| Teraspeed (R) Labs.
| http://www.teraspeed.com
[IBIS Ver]   3.2
[Comment Char] |_char
[File Name]   lm98620.ibs
[File Rev]   3.0
[Source]  Teraspeed (R) Labs.
[Date]   02-17-2009
[Notes]   Quality Check of this IBIS model: Model Passes IBIS Check
   Model parses into ICX IS. Simulation done with Hyperlynx.
   1. MIN TYP MAX information is based on Temprature and Voltage
   characteristics only.
   2. Package data measured using Tektronix IConnect Software.
[Disclaimer]
|(C) Copyright National Semiconductor Corporation 2009
|   All rights reserved
|   National Semiconductor Corporation hereby grants
|the user of this IBIS model a non-exclusive, nontransferable
|license to use this IBIS model under the following terms.
|Before using this IBIS model, the user should read this
|license.  If the user does not accept these terms,  the
|IBIS model should be returned to National within 30 days.
|   The user is granted this license only to use the
|IBIS model and is not granted rights to sell, load, rent,
|lease or license the IBIS model in whole or in part, or in
|modified form to anyone other than user. User may modify
|the IBIS model to suit its specific applications but rights
|to derivative works and such modifications shall belong to
|National.
|   This IBIS model is provided on an "AS IS" basis and
|National makes absolutely no warranty with respect to the
|information contained herein.NATIONAL DISCLAIMS AND CUSTOMER
|WAIVES ALL WARRANTIES, EXPRESS OR IMPLIED, INCLUDING
|WARRANTIES OF MERCHANTABILITY OR FITNESS FOR A PARTICULAR
|PURPOSE. The entire risk as to quality and performance is
|with the Customer. ACCORDINGLY, IN NO EVENT SHALL THE
|COMPANY BE LIABLE FOR ANY DAMAGES, WHETHER IN CONTRACT OR
|TORT,INCLUDING ANY LOST PROFITS OR OTHER INCIDENTAL,
|CONSEQUENTIAL, EXEMPLARY, OR PUNITIVE DAMAGES ARISING OUT
|OF THE USE OR APPLICATION OF THE IBIS model provided in
|this package.Further, National reserves the right to make
|changes without notice to any product herein to improve
|reliability, function, or design. National does not convey
|any license under patent rights or any other intellectual
|property rights, including those of third parties.
|   National is not obligated to provide maintenance or support
|for the licensed IBIS model.
| Use: Teraspeed (R) Labs has licensed Teraspeed (R) AccuModel (tm)
| IBIS models to specific integrated circuit suppliers ("IC Vendors")
| for use and distribution as  follows: Each IC Vendor may use IBIS
| Models, and distribute them to IC Vendor's customers to use solely
| for developing printed circuit board designs. Users of this model may
| modify the IBIS model to suit its specific applications but
| rights to derivative works and such modifications shall belong
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[Copyright]
| This file is the legal property of National Semiconductor and
| Teraspeed Copyright(c) 2009.
| All other rights are reserved.
[Component]   LM98620
[Manufacturer] National Semiconductor
[Package]
| variable   typ   min   max
R_pkg  1.848E-02   1.490E-02   2.216E-02
L_pkg  1.664E-09   1.340E-09   1.990E-09
C_pkg  4.630E-13   3.720E-13   5.590E-13
[Pin] signal_name  model_name  R_pin  L_pin C_pin
1   SHD/HOLD   in_gen   2.216E-02  1.990E-09  5.590E-13
2   VDDD   POWER   2.134E-02  1.920E-09  5.370E-13
3   VSSD   GND   2.060E-02  1.850E-09  5.150E-13
4   CLPIN   in_gen   1.970E-02  1.780E-09  4.930E-13
5   BLKCLP   in_pd   1.890E-02  1.700E-09  4.720E-13
6   AGC_ONB   in_pu   1.800E-02  1.620E-09  4.510E-13
7   OVPB   in_gen   1.720E-02  1.550E-09  4.300E-13
8   MCLK   in_gen   1.640E-02  1.480E-09  4.100E-13
9   GPI1   in_gpi   1.560E-02  1.410E-09  3.910E-13
10  GPI2   in_gpi   1.490E-02  1.340E-09  3.720E-13
11  GPI3   in_gpi   1.490E-02  1.340E-09  3.720E-13
12  GPI4   in_gpi   1.560E-02  1.410E-09  3.910E-13
13  GPI5   in_gpi   1.640E-02  1.480E-09  4.100E-13
14  VSSD   GND   1.720E-02  1.550E-09  4.300E-13
15  VDDD   POWER   1.800E-02  1.620E-09  4.510E-13
16  IBIAS   term   1.890E-02  1.700E-09  4.720E-13
17  VREG1   term   1.970E-02  1.780E-09  4.930E-13
18  VSSD   GND   2.060E-02  1.850E-09  5.150E-13
19  VDDD   POWER   2.134E-02  1.920E-09  5.370E-13
20  VREG2   term   2.216E-02  1.990E-09  5.590E-13
21  TCLK1+   out_lvds   2.216E-02  1.990E-09  5.590E-13
22  TCLK1-   out_lvds   2.134E-02  1.920E-09  5.370E-13
23  TXOUTC1+   out_lvds   2.060E-02  1.850E-09  5.150E-13
24  TXOUTC1-   out_lvds   1.970E-02  1.780E-09  4.930E-13
25  TXOUTB1+   out_lvds   1.890E-02  1.700E-09  4.720E-13
26  TXOUTB1-   out_lvds   1.800E-02  1.620E-09  4.510E-13
27  VREG2   term   1.720E-02  1.550E-09  4.300E-13
28  VSSLVDS   GND   1.640E-02  1.480E-09  4.100E-13
29  TXOUTA1+   out_lvds   1.560E-02  1.410E-09  3.910E-13
30  TXOUTA1-   out_lvds   1.490E-02  1.340E-09  3.720E-13
31  TCLK2+   out_lvds   1.490E-02  1.340E-09  3.720E-13
32  TCLK2-   out_lvds   1.560E-02  1.410E-09  3.910E-13
33  VREG2   term   1.640E-02  1.480E-09  4.100E-13
34  VSSLVDS   GND   1.720E-02  1.550E-09  4.300E-13
35  TXOUTC2+   out_lvds   1.800E-02  1.620E-09  4.510E-13
36  TXOUTC2-   out_lvds   1.890E-02  1.700E-09  4.720E-13
37  TXOUTB2+   out_lvds   1.970E-02  1.780E-09  4.930E-13
38  TXOUTB2-   out_lvds   2.060E-02  1.850E-09  5.150E-13
39  TXOUTA2+   out_lvds   2.134E-02  1.920E-09  5.370E-13
40  TXOUTA2-   out_lvds   2.216E-02  1.990E-09  5.590E-13
41  VSSLVDS   GND   2.216E-02  1.990E-09  5.590E-13
42  VSSLVDS   GND   2.134E-02  1.920E-09  5.370E-13
43  VREG2   term   2.060E-02  1.850E-09  5.150E-13
44  VDDLVDS   POWER   1.970E-02  1.780E-09  4.930E-13
45  VDDLVDS   POWER   1.890E-02  1.700E-09  4.720E-13
46  VREG1   term   1.800E-02  1.620E-09  4.510E-13
47  TESTO_1   out_tri   1.720E-02  1.550E-09  4.300E-13
48  TESTO_0   out_tri   1.640E-02  1.480E-09  4.100E-13
49  RESETB   in_pu   1.560E-02  1.410E-09  3.910E-13
50  SCLK   in_gen   1.490E-02  1.340E-09  3.720E-13
51  SDI   in_gen   1.490E-02  1.340E-09  3.720E-13
52  SENB   in_pu   1.560E-02  1.410E-09  3.910E-13
53  SDO   out_tri   1.640E-02  1.480E-09  4.100E-13
54  VDDD   POWER   1.720E-02  1.550E-09  4.300E-13
55  VSSD   GND   1.800E-02  1.620E-09  4.510E-13
56  VSSA   GND   1.890E-02  1.700E-09  4.720E-13
57  VREF   term   1.970E-02  1.780E-09  4.930E-13
58  VDDA   POWER   2.060E-02  1.850E-09  5.150E-13
59  VREFTOUT   term   2.134E-02  1.920E-09  5.370E-13
60  VREFBOUT   term   2.216E-02  1.990E-09  5.590E-13
61  VREFBIN2   term   2.216E-02  1.990E-09  5.590E-13
62  VREFTIN2   term   2.134E-02  1.920E-09  5.370E-13
63  VREFBIN1   term   2.060E-02  1.850E-09  5.150E-13
64  VREFTIN1   term   1.970E-02  1.780E-09  4.930E-13
65  VSSA   GND   1.890E-02  1.700E-09  4.720E-13
66  OSR1   term   1.800E-02  1.620E-09  4.510E-13
67  VDDA   POWER   1.720E-02  1.550E-09  4.300E-13
68  OSR2   term   1.640E-02  1.480E-09  4.100E-13
69  VSSA   GND   1.560E-02  1.410E-09  3.910E-13
70  OSG1   term   1.490E-02  1.340E-09  3.720E-13
71  VDDA   POWER   1.490E-02  1.340E-09  3.720E-13
72  OSG2   term   1.560E-02  1.410E-09  3.910E-13
73  VSSA   GND   1.640E-02  1.480E-09  4.100E-13
74  OSB1   term   1.720E-02  1.550E-09  4.300E-13
75  VDDA   POWER   1.800E-02  1.620E-09  4.510E-13
76  OSB2   term   1.890E-02  1.700E-09  4.720E-13
77  VSSA   GND   1.970E-02  1.780E-09  4.930E-13
78  VCLP_EXT   POWER   2.060E-02  1.850E-09  5.150E-13
79  VLCP_INT   term   2.134E-02  1.920E-09  5.370E-13
80  SHP/SAMPLE in_gen   2.216E-02  1.990E-09  5.590E-13
[Diff Pin] inv_pin vdiff tdelay_typ tdelay_min tdelay_max
21  22  NA  NA  NA  NA
23  24  NA  NA  NA  NA
25  26  NA  NA  NA  NA
29  30  NA  NA  NA  NA
31  32  NA  NA  NA  NA
35  36  NA  NA  NA  NA
37  38  NA  NA  NA  NA
39  40  NA  NA  NA  NA
[Model] term
Model_type Terminator
C_comp   0  0  0
| variable   typ   min   max
[Voltage Range]   3.30000V  3.00000V  3.60000V
[POWER Clamp Reference]  3.30000V  3.00000V  3.60000V
[GND Clamp Reference]   0.00000V  0.00000V  0.00000V
[Temperature Range]   25   70   0
| Models and submodels in the file (7): in_gen (Input), in_gpi (Input), in_pd (Input), in_pu (Input), out_lvds (Output), out_tri (3-state), term (Terminator)
